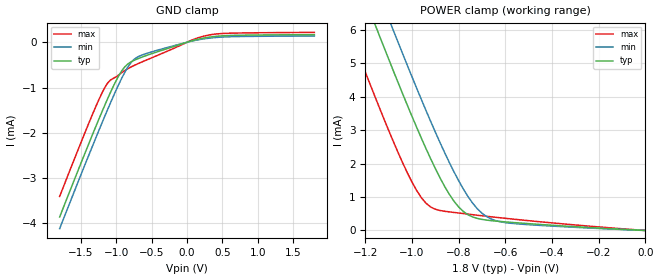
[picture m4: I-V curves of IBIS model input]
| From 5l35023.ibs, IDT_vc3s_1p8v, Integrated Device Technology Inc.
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|   Model INPUT
[Model]  input
Model_type Input
Vinl =   0.6300V
Vinh =   1.1700V
C_comp   2.0000pF   1.5000pF   2.5000pF
[Temperature Range]   55.0000   0.1050k   -40.0000
[Voltage Range]   1.8000V   1.7100V   1.8900V
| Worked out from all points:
|   GND clamp passes 1 mA (typ) near -1.05 V on its own axis
|   POWER clamp passes 1 mA (typ) near -0.83 V on its own axis
[GND_clamp]
|Voltage   I(typ)   I(min)   I(max)
-1.8V     -3.862mA   -4.119mA   -3.407mA
-1.36V    -2.134mA   -2.388mA   -1.684mA
-1.16V    -1.385mA   -1.627mA   -995.8uA
-1.08V    -1.103mA   -1.334mA   -833.5uA
-920mV    -626.6uA   -787.2uA   -668.4uA
-800mV    -441.7uA   -466.4uA   -553.2uA
-720mV    -379.9uA   -345.1uA   -492.5uA
-240mV    -120.3uA   -99.19uA   -171.4uA
80mV      37.24uA    29.96uA    55.25uA
320mV     113.6uA    91.83uA    162.7uA
640mV     151.2uA    123.4uA    201.4uA
1.8V      168.3uA    138.7uA    218uA
[POWER_clamp]
|Voltage   I(typ)   I(min)   I(max)
-1.8V     18.02mA    19.18mA    15.95mA
-1.28V    8.37mA     9.596mA    6.191mA
-1.26V    8.004mA    9.229mA    5.825mA
-1.16V    6.193mA    7.413mA    4.031mA
-1.14V    5.836mA    7.054mA    3.681mA
-1.08V    4.779mA    5.987mA    2.664mA
-1V       3.416mA    4.597mA    1.449mA
-940mV    2.451mA    3.59mA     816.2uA
-820mV    875.8uA    1.754mA    539.1uA
-700mV    331uA      515.3uA    439.7uA
-580mV    245.4uA    217.8uA    348.9uA
0V        1.911pA    4.287pA    1.89pA
